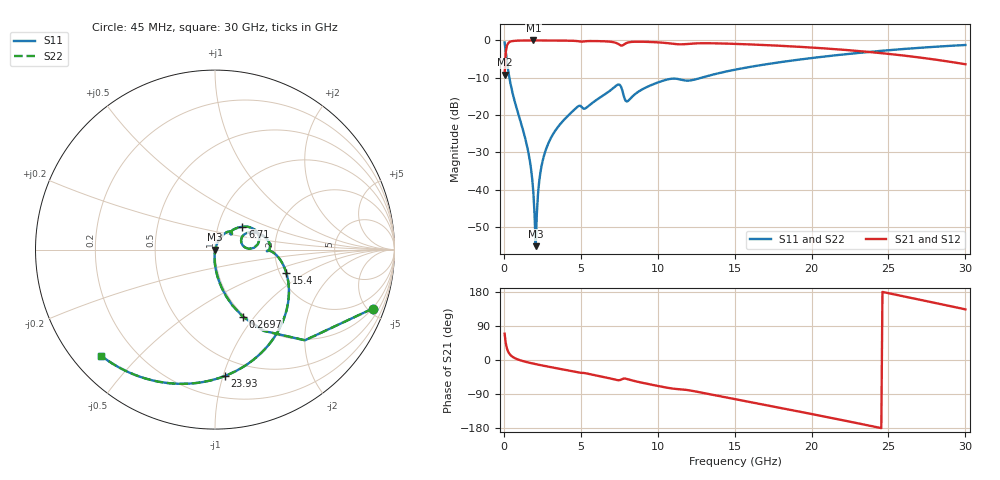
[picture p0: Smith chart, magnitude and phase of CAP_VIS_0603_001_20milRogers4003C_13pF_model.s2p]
! S-parameter model data by Modelithics Inc.  support@modelithics.com  813-866-6335  Tampa FL USA
! S-Parameter data specifications:
! Substrate: 20-mil Rogers 4003C, substrate thickness, H=0.508mm, Dielectric constant, Er=3.75
! PCB Mounting Pad Footprint: Pad width, PadW=0.90mm , Pad length, PadL=1.00mm , Pad gap, PadG (edge-to-edge)=1.00mm , Reference planes=3.0mm apart
! Created Wed Nov 18 13:26:32 2015
# hz S ma R 50
! 2 Port Network Data from SP1.SP block
! freq  magS11  angS11  magS21  angS21  magS12  angS12  magS22  angS22
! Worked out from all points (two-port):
!   401 points, 45 MHz to 30 GHz, reference 50 ohm
!   highest |S21| = -0.02 dB at 1.917 GHz (marker M1); lowest = -9.2 dB at 45 MHz (marker M2)
!   |S21| within 3 dB of the highest: 122.4 MHz to 23.51 GHz (23.39 GHz wide, 198 % of centre)
!   lowest |S11| = -55.2 dB at 2.067 GHz (marker M3), VSWR 1.00, Z = 50.2 - j0.0155 ohm
!   |S11| at or under -10 dB: 355.5 MHz to 12.85 GHz (12.49 GHz wide, 189 % of centre)
!   |S22| runs from -55.2 to -0.6 dB; largest |S21 - S12| = 0
!   S11 on the Smith chart (normalised r, x): 45 MHz: 0.98, -5.36; 269.7 MHz: 0.98, -0.88; 6.71 GHz: 1.31, +0.35; 15.4 GHz: 2.17, -0.69; 23.93 GHz: 0.36, -1.01; 30 GHz: 0.08, -0.39
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4.5e7  0.9381 -20.5  0.3463 69.5  0.3463 69.5  0.9381 -20.5
2.696625e8  0.406 -67.4  0.9132 22.5  0.9132 22.5  0.406 -67.4
5.692125e8  0.1942 -81.5  0.98 8.2  0.98 8.2  0.1942 -81.5
1.54275e9  0.03514 -93.7  0.9978 -6.1  0.9978 -6.1  0.03514 -93.7
1.767412e9  0.01865 -93.3  0.9981 -8.3  0.9981 -8.3  0.01865 -93.3
1.917188e9  0.008983 -88.9  0.9981 -9.6  0.9981 -9.6  0.008983 -88.9
2.066962e9  0.001744 -5.1  0.9981 -10.9  0.9981 -10.9  0.001744 -5.1
2.216738e9  0.008777 66.0  0.998 -12.2  0.998 -12.2  0.008777 66.0
2.4414e9  0.02045 70.6  0.9977 -14.0  0.9977 -14.0  0.02045 70.6
2.890725e9  0.04186 69.5  0.9968 -17.6  0.9968 -17.6  0.04186 69.5
3.864262e9  0.08429 62.8  0.9932 -25.2  0.9932 -25.2  0.08429 62.8
5.062462e9  0.1277 42.6  0.9619 -33.8  0.9619 -33.8  0.1277 42.6
6.709988e9  0.1985 39.8  0.9678 -46.8  0.9678 -46.8  0.1985 39.8
7.458862e9  0.2569 18.3  0.8884 -53.4  0.8884 -53.4  0.2569 18.3
8.057962e9  0.1538 19.1  0.9359 -50.7  0.9359 -50.7  0.1538 19.1
1.007992e10  0.2762 16.6  0.9398 -69.1  0.9398 -69.1  0.2762 16.6
1.50225e10  0.4047 -15.5  0.8983 -103.4  0.8983 -103.4  0.4047 -15.5
1.539694e10  0.4187 -18.2  0.8928 -106.3  0.8928 -106.3  0.4187 -18.2
2.003996e10  0.5812 -53.9  0.8008 -142.8  0.8008 -142.8  0.5812 -53.9
2.393411e10  0.7064 -85.6  0.6936 -174.7  0.6936 -174.7  0.7064 -85.6
2.505742e10  0.7401 -95.0  0.6577 175.9  0.6577 175.9  0.7401 -95.0
3e10  0.8675 -137.1  0.4788 133.7  0.4788 133.7  0.8675 -137.1
